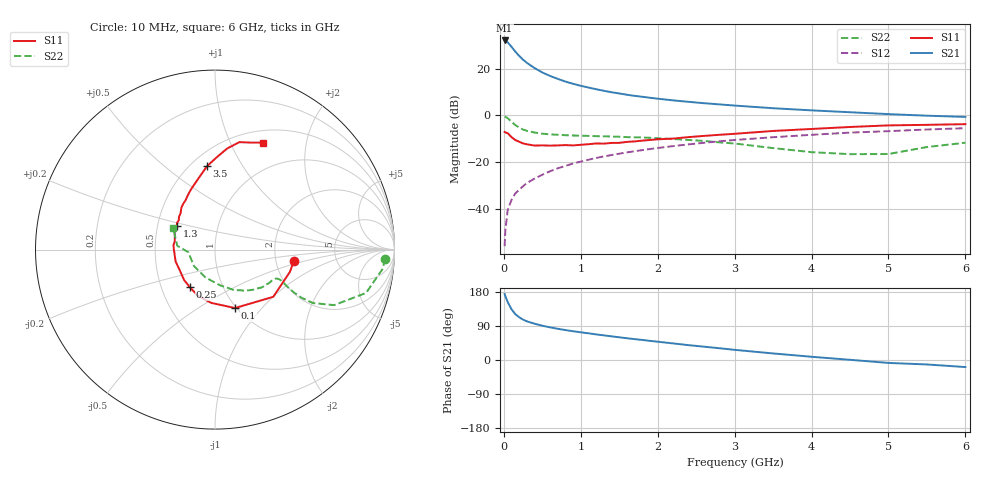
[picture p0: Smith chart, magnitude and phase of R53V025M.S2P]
! SIEMENS Small Signal Semiconductors
! BFR183
! Si NPN RF Bipolar Junction Transistor in SOT23
! VCE = 3 V  IC = 25 mA
! Common Emitter S-Parameters:  May  1996
# GHz  S  MA  R  50
!  f  S11  S21  S12  S22
! GHz  MAG  ANG  MAG  ANG  MAG  ANG  MAG  ANG
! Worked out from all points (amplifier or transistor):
!   36 points, 10 MHz to 6 GHz, reference 50 ohm
!   highest |S21| = 32.1 dB at 10 MHz (marker M1)
!   |S21| within 3 dB of that: start of sweep to 106.2 MHz
!   unconditionally stable (mu >= 1): 472.8 MHz to 2.336 GHz
!   at 250 MHz: K = 0.86, MSG = 27.1 dB, |S12| = -30.3 dB
!   at 1.4 GHz: K = 1.05, MAG = 12.1 dB, |S12| = -16.9 dB
!   at 6 GHz: K = 0.90, MSG = 2.4 dB, |S12| = -5.4 dB
!   S11 on the Smith chart (normalised r, x): 10 MHz: 2.51, -0.41; 100 MHz: 0.98, -0.73; 250 MHz: 0.70, -0.31; 1.3 GHz: 0.63, +0.18; 3.5 GHz: 0.60, +0.71; 6 GHz: 0.64, +1.33
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0.01  0.4435 -8.5  40.28 174.0  0.0016 84.3  0.9509 -3.1
0.02  0.4354 -16.6  39.76 168.2  0.0035 81.5  0.938 -6.8
0.05  0.4179 -39.0  36.73 153.0  0.0095 77.8  0.8756 -16.0
0.1  0.3442 -71.1  29.38 133.8  0.0157 72.4  0.7323 -25.0
0.15  0.2976 -94.1  23.17 120.8  0.0216 68.6  0.6222 -28.6
0.2  0.2741 -110.4  18.82 112.7  0.0259 69.9  0.551 -29.1
0.25  0.2519 -124.0  15.63 106.5  0.0306 69.8  0.5011 -28.5
0.3  0.2419 -135.2  13.35 102.0  0.0358 71.2  0.4698 -27.8
0.4  0.2273 -150.5  10.31 95.8  0.0448 72.4  0.4314 -26.2
0.5  0.2292 -163.2  8.323 90.5  0.054 73.0  0.4083 -25.2
0.6  0.2266 -171.6  7.027 86.2  0.064 72.9  0.3953 -24.8
0.7  0.2288 -179.4  6.074 82.4  0.0739 73.0  0.3866 -24.9
0.8  0.2326 173.8  5.323 79.0  0.0835 72.1  0.3788 -25.2
0.9  0.229 167.9  4.763 75.9  0.0938 71.5  0.3734 -25.6
1.1  0.243 157.5  3.958 70.4  0.1132 70.3  0.3658 -27.8
1.3  0.25 148.2  3.371 65.0  0.1332 68.5  0.358 -29.9
1.7  0.279 133.4  2.631 55.1  0.1719 64.6  0.3411 -35.6
2.2  0.3203 120.8  2.105 43.8  0.2212 58.9  0.3151 -44.8
3.5  0.4667 95.5  1.43 17.3  0.3427 42.2  0.2007 -82.0
4.5  0.5676 83.1  1.173 0.5  0.43 29.3  0.1488 -141.7
5.5  0.6306 70.9  0.99 -11.8  0.5012 17.5  0.2113 174.3
6  0.6527 66.0  0.932 -18.6  0.5345 9.9  0.2613 152.9
